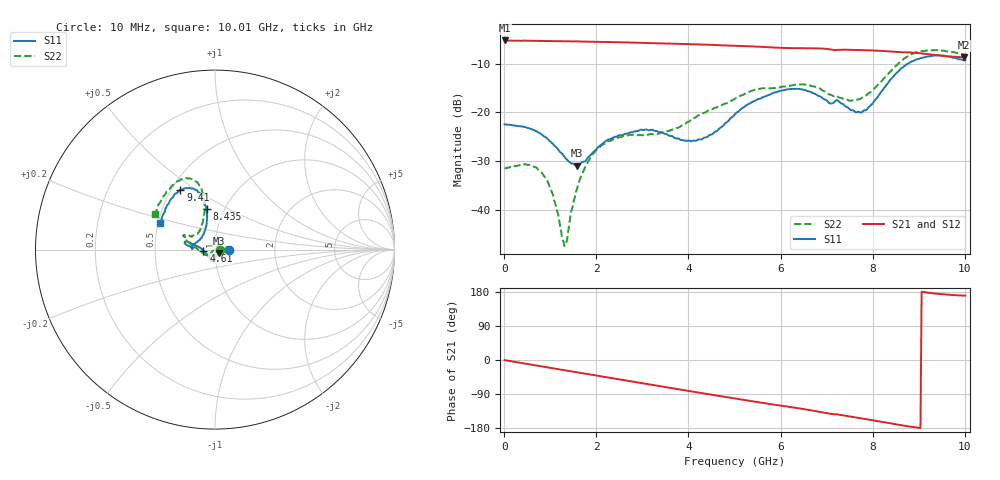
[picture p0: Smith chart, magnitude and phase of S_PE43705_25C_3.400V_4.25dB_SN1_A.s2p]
! Device ID: PE43705
! Serial: 1
! Insertion: A
! Impedance: 50 ohm
! Temp: 25C
! VDD: 3.400V
! Attenuation Step: 4.25dB
#  Hz  S  RI  R  50
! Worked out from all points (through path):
!   401 points, 10 MHz to 10.01 GHz, reference 50 ohm
!   highest |S21| = -5.28 dB at 10 MHz (marker M1); lowest = -8.7 dB at 9.985 GHz (marker M2)
!   group delay of S21, straight-line fit = 54.3 ps
!   lowest |S11| = -30.9 dB at 1.585 GHz (marker M3), VSWR 1.06, Z = 52 - j2.13 ohm
!   |S11| at or under -10 dB: start of sweep to 8.77 GHz
!   |S22| runs from -47.3 to -7.2 dB; largest |S21 - S12| = 0.0049
!   S11 on the Smith chart (normalised r, x): 10 MHz: 1.16, -0.00; 4.61 GHz: 0.88, -0.01; 8.435 GHz: 0.83, +0.39; 9.41 GHz: 0.56, +0.43; 10.01 GHz: 0.51, +0.17
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1e7  0.0758 -0.000311  0.5448 -0.0028  0.5451 -0.0024  0.0272 2.58e-05
5.35e8  0.068 0.0129  0.5296 -0.1061  0.5299 -0.1058  0.0235 0.0172
8.35e8  0.0574 0.0118  0.514 -0.1615  0.5139 -0.1611  0.0158 0.0176
1.06e9  0.0474 0.00551  0.4965 -0.2019  0.4968 -0.2016  0.00782 0.0121
1.31e9  0.0349 -0.00566  0.4758 -0.2443  0.4759 -0.2441  -0.00269 0.00335
1.585e9  0.02 -0.0204  0.447 -0.2888  0.4472 -0.2887  -0.014 -0.00927
1.685e9  0.0156 -0.0268  0.4359 -0.3041  0.4359 -0.304  -0.0188 -0.0141
1.935e9  0.00466 -0.0393  0.4052 -0.3403  0.4053 -0.3399  -0.0292 -0.0243
2.235e9  -0.00482 -0.0519  0.3641 -0.3791  0.3643 -0.3789  -0.0382 -0.0329
3.36e9  -0.0203 -0.06  0.1842 -0.4748  0.1849 -0.4743  -0.0536 -0.029
4.085e9  -0.04 -0.0321  0.0589 -0.4944  0.0595 -0.4942  -0.0862 -0.00743
4.61e9  -0.0641 -0.00638  -0.0324 -0.4878  -0.0311 -0.4876  -0.1117 0.0133
5.01e9  -0.0944 0.0173  -0.0965 -0.471  -0.0959 -0.4712  -0.1352 0.0308
5.985e9  -0.1596 0.0455  -0.2295 -0.3966  -0.2277 -0.3971  -0.1669 0.0693
6.685e9  -0.1569 0.0252  -0.311 -0.3291  -0.3109 -0.3285  -0.1674 0.0797
7.71e9  -0.0788 0.063  -0.3885 -0.1957  -0.3875 -0.1968  -0.0843 0.1075
8.36e9  -0.0445 0.2049  -0.4098 -0.0983  -0.4085 -0.1001  -0.0589 0.2499
8.435e9  -0.0472 0.225  -0.4096 -0.086  -0.4087 -0.0878  -0.0596 0.2721
8.86e9  -0.0955 0.3204  -0.4081 -0.0239  -0.4052 -0.0259  -0.1107 0.3814
9.41e9  -0.1927 0.3313  -0.3828 0.0361  -0.3815 0.0355  -0.2097 0.381
9.985e9  -0.2982 0.1599  -0.3612 0.0646  -0.3623 0.0645  -0.3285 0.2091
1.001e10  -0.3058 0.1506  -0.3625 0.0657  -0.3643 0.065  -0.3361 0.198
